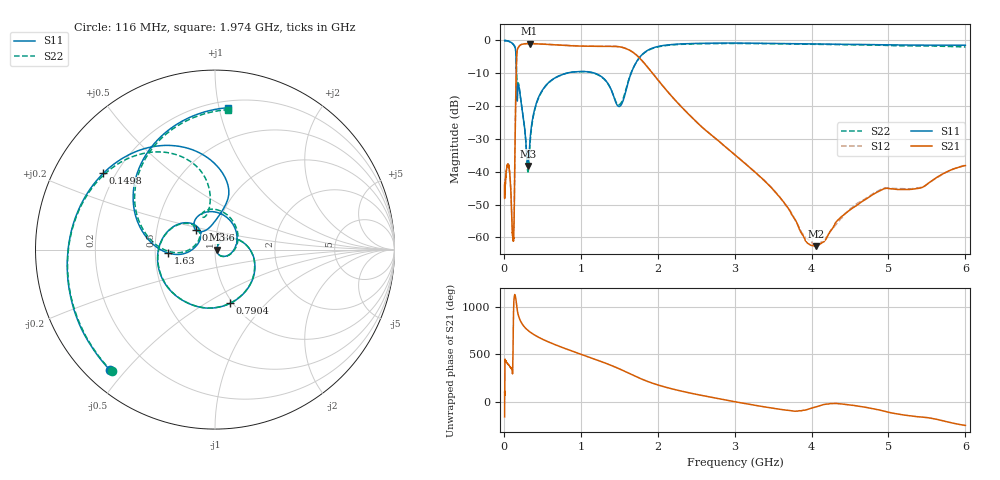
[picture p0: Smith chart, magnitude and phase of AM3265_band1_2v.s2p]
!Agilent Technologies,E8364B,MY43040894,A.07.50.67
!Agilent E8364B: A.07.50.67
!Date: Friday, May 09, 2025 07:14:08
!Correction: S11(Full 2 Port(1,2))
!S21(Full 2 Port(1,2))
!S12(Full 2 Port(1,2))
!S22(Full 2 Port(1,2))
!S2P File: Measurements: S11, S21, S12, S22:Log Frequency Sweep
# Hz S  dB  R 50
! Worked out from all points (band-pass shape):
!   3201 points, 10 MHz to 6 GHz, reference 50 ohm
!   highest |S21| = -0.97 dB at 335.3 MHz (marker M1); lowest = -62.7 dB at 4.055 GHz (marker M2)
!   |S21| within 3 dB of the highest: 169.5 MHz to 1.699 GHz (1.53 GHz wide, 164 % of centre)
!   lowest |S11| = -38.2 dB at 311.4 MHz (marker M3), VSWR 1.02, Z = 51.2 - j0.0128 ohm
!   |S11| at or under -10 dB: 162.6 MHz to 812 MHz (649.4 MHz wide, 133 % of centre); 1.184 GHz to 1.654 GHz (469.4 MHz wide, 33.1 % of centre)
!   |S22| runs from -40.1 to 0.0 dB; largest |S21 - S12| = 0.012
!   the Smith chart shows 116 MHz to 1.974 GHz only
!   S11 on the Smith chart (normalised r, x): 116 MHz: 0.07, -0.45; 149.8 MHz: 0.15, +0.30; 178.6 MHz: 0.79, +0.17; 790.4 MHz: 0.97, -0.65; 1.63 GHz: 0.59, -0.02; 1.974 GHz: 0.25, +1.06
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1e7  0.00 -9.4  -43.88 -155.7  -44.11 135.6  -0.07 -9.5
2.908064e7  -0.06 -27.2  -40.43 64.7  -40.18 63.4  -0.06 -27.2
8.439949e7  -0.43 -85.9  -42.75 5.5  -42.98 6.8  -0.46 -85.8
1.15979e8  -1.01 -131.3  -59.42 4.1  -58.55 136.6  -1.02 -130.4
1.315449e8  -1.44 -161.3  -57.39 -8.1  -55.15 -40.7  -1.43 -159.2
1.497977e8  -2.45 145.6  -24.26 32.5  -24.30 32.5  -2.36 151.8
1.786094e8  -16.42 134.6  -2.56 -133.7  -2.53 -133.6  -13.95 111.7
2.44949e8  -21.95 -23.5  -1.11 92.6  -1.07 92.5  -21.88 -24.4
3.113553e8  -38.24 -0.6  -0.98 34.3  -0.94 34.2  -39.98 -9.0
3.352576e8  -31.96 54.3  -0.97 18.7  -0.93 18.7  -33.33 60.4
7.123273e8  -10.85 -52.8  -1.39 -132.2  -1.35 -132.2  -10.86 -53.2
7.903593e8  -10.14 -74.2  -1.49 -156.3  -1.45 -156.3  -10.15 -74.8
1.193076e9  -10.08 178.5  -1.80 86.3  -1.77 86.3  -10.15 177.7
1.629682e9  -11.66 -175.8  -2.91 -59.6  -2.89 -59.6  -11.50 -178.5
1.974456e9  -2.00 84.7  -11.21 -174.2  -11.18 -174.2  -2.12 84.8
2.067357e9  -1.55 62.7  -13.88 163.2  -13.86 163.1  -1.67 63.0
2.455151e9  -0.92 -11.1  -23.70 87.6  -23.68 87.6  -1.05 -10.5
2.96862e9  -0.79 -90.1  -34.15 7.1  -34.16 6.9  -0.90 -90.3
3.518433e9  -0.90 -166.6  -45.94 -68.4  -45.81 -68.4  -1.00 -168.4
4.054987e9  -1.07 123.1  -62.68 -52.7  -62.29 -49.7  -1.18 120.7
5.002045e9  -1.35 4.2  -45.12 -109.4  -44.92 -109.8  -1.54 4.7
6e9  -1.45 -115.3  -38.11 112.5  -38.02 112.7  -1.97 -111.1
